//DB988.AWL
// ***************************************************************************

DATA_BLOCK "XC_RASTA_SR"
TITLE = Cross Coupling ASTA

AUTHOR: 	SIEMENS
FAMILY: 	SISTARS7
NAME:		XCASTA
VERSION: 	4.02

//$NOW_HOW_PROTECT

//
// Datum		Name			Aktion
// ----------------------------------------------------------------------------
// 25.06.99 	Mahler		Neu

  STRUCT

	iType			: INT		:= 1;
   	iOffset 		: INT  	:= 20;
   	iLen 			: INT  	:= 12;


//#IF Default
   	iMax 			: INT  	:= 64;
   	iAct 			: INT  	:= 64;
//#ENDIF

//#IF Special
// 	iMax 			: INT  	:= %TA%;
// 	iAct 			: INT  	:= %TA%;
//#ENDIF
	iRecord		: INT;

	ab			: ARRAY [1..8] OF BYTE;

//#IF Default
	au			: ARRAY [1..96] OF "XC_ASTA_UDT";
//#ENDIF

//#IF Special
//	au			: ARRAY [1..%TA%] OF "XC_ASTA_UDT";
//#ENDIF


END_STRUCT ;

BEGIN

END_DATA_BLOCK

